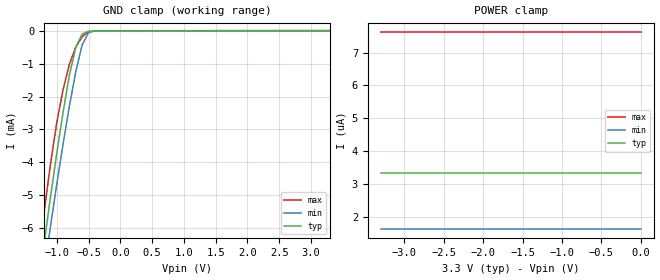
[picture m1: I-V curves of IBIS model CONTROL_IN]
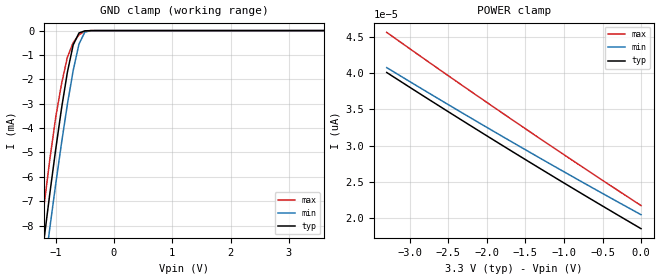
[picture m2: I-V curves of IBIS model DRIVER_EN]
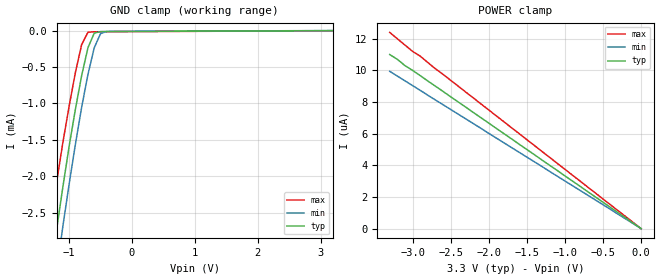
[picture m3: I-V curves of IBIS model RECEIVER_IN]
|   Texas Instruments Incorporated
|   Data Transmissions Products
|   IBIS Model for SN65LVDS22
|   16D SOIC Package
[IBIS Ver]   3.2
[Comment char]   |_char
[File name]   lvds22a.ibs
[File Rev]   2.0
[Date]   19Feb03
[Source]   File originated at Texas Instruments Incorporated.
   Data Transmission Products Group.
|   This model was updated to provide C_comp, mins and maxs
[Notes]
[Disclaimer]
(C) Copyright Texas Instruments Incorporated 2003
   All rights reserved
  Texas Instruments Incorporated hereby grants the user of this IBIS
model a non-exclusive, nontransferable license to use this IBIS model
under the following terms.  Before using this IBIS model, the user
should read this license.  If the user does not accept these terms,
the IBIS model should be returned to Texas Instruments within 30 days.
  The user is granted this license only to use the IBIS model and
is not granted rights to sell, load, rent, lease or license the IBIS
model in whole or in part, or in modified form to anyone other than
user.  User may modify the IBIS model to suit its specific applications
but rights to derivative works and such modifications shall belong to
Texas Instruments.
  This IBIS model is provided on an "AS IS" basis and Texas Instruments
makes absolutely no warranty with respect to the information contained
herein.  TEXAS INSTRUMENTS DISCLAIMS AND CUSTOMER WAIVES ALL WARRANTIES,
EXPRESS OR IMPLIED, INCLUDING WARRANTIES OF MERCHANTABILITY OR FITNESS
FOR A PARTICULAR PURPOSE. The entire risk as to quality and performance
is with the Customer. ACCORDINGLY, IN NO EVENT SHALL THE COMPANY BE LIABLE
FOR ANY DAMAGES, WHETHER IN CONTRACT OR TORT,INCLUDING ANY LOST PROFITS
OR OTHER INCIDENTAL, CONSEQUENTIAL, EXEMPLARY, OR PUNITIVE DAMAGES ARISING
OUT OF THE USE OR APPLICATION OF THE IBIS model provided in this package.
Further, Texas Instruments reserves the right to discontinue or make changes
without notice to any product herein to improve reliability, function, or
design. Texas Instruments does not convey any license under patent rights
or any other intellectual property rights, including those of third parties.
Contact Texas Instruments at ATTN:DATA TRANSMISSIONS
Thomas Fisher 8505 Forest Lane, M/S 8710, Dallas, TX 75243-4136
[Copyright]   Copyright 2003, Texas Instruments, All Rights Reserved
[Component]   LVDS22D
[Manufacturer]  Texas Instruments Incorporated
[Package]
|   typ   min   max
R_pkg   0.035   0.030   0.040
L_pkg   2.181nH   1.231nH   3.257nH
C_pkg   0.322pF   0.163pF   0.546pF
[Pin]   signal_name   model_name   R_pin   L_pin   C_pin
1   1B   RECEIVER_IN   0.040   3.251n   0.546p
2   1A   RECEIVER_IN   0.039   2.561n   0.393p
3   S0   CONTROL_IN   0.030   1.681n   0.186p
4   1DE   DRIVER_EN   0.030   1.231n   0.163p
5   S1   CONTROL_IN   0.030   1.231n   0.163p
6   2A   RECEIVER_IN   0.030   1.681n   0.186p
7   2B   RECEIVER_IN   0.039   2.564n   0.393p
8   GND   GND   0.040   3.257n   0.545p
9   GND   GND   0.040   3.247n   0.546p
10   2Y   DRIVER_OUT   0.039   2.558n   0.394p
11   2Z   DRIVER_OUT   0.030   1.681n   0.187p
12   2DE   DRIVER_EN   0.030   1.231n   0.163p
13   1Z   DRIVER_OUT   0.030   1.231n   0.163p
14   1Y   DRIVER_OUT   0.030   1.681n   0.187p
15   VCC   POWER   0.039   2.558n   0.394p
16   VCC   POWER   0.040   3.246n   0.546p
[Diff_pin]   inv_pin   vdiff   tdelay_typ   tdelay_min   tdelay_max
| The 'xY' pin is Diff_pin and the 'xZ' pin is the inv_pin
2   1   0.100   0 0 0
6   7   0.100   0 0 0
10   11   0.000   0 0 0
14   13   0.000   0 0 0
| Models and submodels in the file (4): CONTROL_IN (Input), DRIVER_EN (Input), RECEIVER_IN (Input), DRIVER_OUT (3-state)
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|   Control Input MODEL
[Model]   CONTROL_IN
Model_type   Input
|Signals   S0,S1
Vinh = 2.0
Vinl = 0.8
|   typ   min   max
C_comp   1.11pF   1.03pF   1.21pF
|   typ   min   max
[Temperature Range]   25.0   -40   85
[Voltage range]   3.3V   3.0V   3.6V
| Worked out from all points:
|   GND clamp passes 1 mA (typ) near -0.76 V on its own axis
[GND_clamp]
|   Voltage   I(typ)   I(min)   I(max)
-3.6V     -49.2mA    -48.3mA    -50.4mA
-1.3V     -7.95mA    -8.69mA    -7.06mA
-1.2V     -6.49mA    -7.31mA    -5.53mA
-1.1V     -5.08mA    -5.97mA    -4.08mA
-1V       -3.73mA    -4.67mA    -2.79mA
-900mV    -2.47mA    -3.44mA    -1.79mA
-800mV    -1.34mA    -2.28mA    -1.01mA
-700mV    -493uA     -1.24mA    -495uA
-600mV    -98.5uA    -429uA     -177uA
-500mV    -13.3uA    -53.4uA    -28.7uA
-400mV    -2.29uA    -3.52uA    -4.22uA
3.3V      3.34uA     1.63uA     7.62uA
[Power_clamp]
| Note that the[POWER_clamp]voltage table is referenced to Vcc
| and is calculated using Vtable=Vcc - Vmeasured.
|   Voltage   I(typ)   I(min)   I(max)
-3.3V     3.34uA     1.63uA     7.62uA
-3.2V     3.34uA     1.63uA     7.62uA
-3.1V     3.34uA     1.63uA     7.62uA
0V        3.34uA     1.63uA     7.62uA
|   Driver Enable  MODEL
[Model]   DRIVER_EN
Model_type   Input
|Signals   1DE, 2DE
Vinh = 2.0
Vinl = 0.8
|   typ   min   max
C_comp   0.99pF   0.93pF   1.05pF
|   typ   min   max
[Temperature Range]   25.0   -40   85
[Voltage range]   3.3V   3.0V   3.6V
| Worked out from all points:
|   GND clamp passes 1 mA (typ) near -0.74 V on its own axis
[GND_clamp]
|   Voltage   I(typ)   I(min)   I(max)
-3.6V     -70.2mA    -71.2mA    -69.9mA
-1.3V     -10.5mA    -11.9mA    -9.2mA
-1.2V     -8.57mA    -9.95mA    -7.19mA
-1.1V     -6.68mA    -8.09mA    -5.28mA
-1V       -4.88mA    -6.31mA    -3.57mA
-900mV    -3.2mA     -4.62mA    -2.19mA
-800mV    -1.72mA    -3.04mA    -1.1mA
-700mV    -589uA     -1.64mA    -495uA
-600mV    -99uA      -551uA     -174uA
-500mV    -11.7uA    -64.1uA    -26.5uA
-400mV    -1.54uA    -3.62uA    -2.66uA
3.6V      20.5pA     24pA       21.8pA
[Power_clamp]
| Note that the[POWER_clamp]voltage table is referenced to Vcc
| and is calculated using Vtable=Vcc - Vmeasured.
|   Voltage   I(typ)   I(min)   I(max)
-3.3V     40.1pA     40.77pA    45.62pA
-2.5V     34.69pA    35.66pA    39.64pA
-1.6V     28.75pA    30.07pA    33.07pA
0V        18.59pA    20.51pA    21.77pA
|   Receiver Input MODEL
[Model]   RECEIVER_IN
Model_type   Input
|Signals   1A,1B,2A,2B
Vinh = 2.0
Vinl = 0.8
|   typ   min   max
C_comp   2.42pF   2.35pF   2.48pF
|   typ   min   max
[Temperature Range]   25.0   -40   85
[Voltage range]   3.3V   3.0V   3.6V
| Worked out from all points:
|   GND clamp passes 1 mA (typ) near -0.88 V on its own axis
[GND_clamp]
|   Voltage   I(typ)   I(min)   I(max)
-3.6V     -26.4mA    -28.3mA    -23.8mA
-1.4V     -4.02mA    -4.68mA    -3.27mA
-1.3V     -3.36mA    -3.98mA    -2.66mA
-1.2V     -2.74mA    -3.32mA    -2.09mA
-1.1V     -2.15mA    -2.69mA    -1.54mA
-900mV    -1.08mA    -1.56mA    -575uA
-800mV    -616uA     -1.05mA    -191uA
-700mV    -234uA     -600uA     -22.8uA
-600mV    -34.5uA    -235uA     -15.8uA
-500mV    -13.2uA    -41uA      -15.4uA
-400mV    -12.3uA    -11.7uA    -15uA
3.2V      -333nA     602nA      -1.5uA
[Power_clamp]
| Note that the[POWER_clamp]voltage table is referenced to Vcc
| and is calculated using Vtable=Vcc - Vmeasured.
|   Voltage   I(typ)   I(min)   I(max)
-3.3V     11uA       9.94uA     12.4uA
-3V       10uA       9.04uA     11.2uA
-2.9V     9.67uA     8.74uA     10.9uA
-2.7V     9uA        8.13uA     10.1uA
0V        7.64pA     11.4pA     9.08pA
